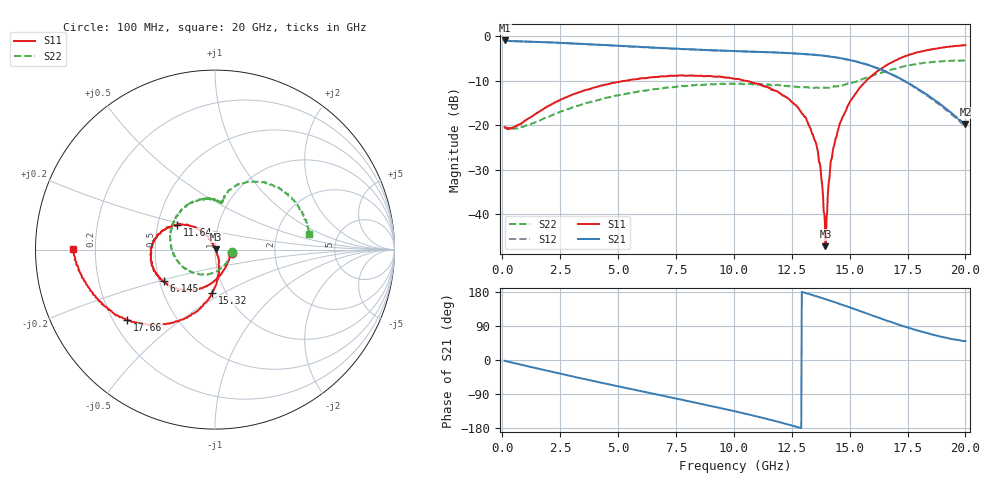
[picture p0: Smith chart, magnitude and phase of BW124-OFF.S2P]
!  2-Port S-parameters saved by WinCal
! VAR MeasName=S-Parameters (CALIBRATED_DATA) read from VNA (N5244A)
! VAR MeasDate=9/14/2012 3:38:30 PM
! VAR NAME=126015-1
! VAR FILENAME=126015-1.S2P
! VAR DATE=9/14/2012 3:38:30 PM
! VAR PHYS_PORTS=1,2
# Hz S MA R 50
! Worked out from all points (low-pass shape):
!   801 points, 100 MHz to 20 GHz, reference 50 ohm
!   highest |S21| = -0.96 dB at 100 MHz (marker M1); lowest = -19.7 dB at 20 GHz (marker M2)
!   |S21| within 3 dB of the highest: start of sweep to 12.9 GHz
!   lowest |S11| = -47.1 dB at 13.96 GHz (marker M3), VSWR 1.01, Z = 50.3 + j0.312 ohm
!   |S11| at or under -10 dB: start of sweep to 5.33 GHz; 10.42192 GHz to 10.4249 GHz (2.98 MHz wide, 0.0286 % of centre); 10.49 GHz to 15.71 GHz (5.216 GHz wide, 39.8 % of centre)
!   |S22| runs from -20.9 to -5.4 dB; largest |S21 - S12| = 0.012
!   S11 on the Smith chart (normalised r, x): 100 MHz: 1.21, -0.04; 6.145 GHz: 0.53, -0.21; 11.64 GHz: 0.63, +0.18; 15.32 GHz: 0.87, -0.44; 17.66 GHz: 0.25, -0.33; 20 GHz: 0.12, +0.00
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1e8  0.09527 -10.2  0.8952 -2.1  0.8914 -2.2  0.09492 -9.2
1.692e9  0.1474 -79.4  0.8581 -24.9  0.8576 -24.9  0.1153 -79.2
3.43325e9  0.2397 -113.7  0.821 -48.7  0.8177 -48.8  0.1715 -129.0
6.144625e9  0.3366 -148.4  0.7532 -84.1  0.7519 -83.9  0.2456 175.9
6.741625e9  0.3505 -155.6  0.7403 -91.8  0.738 -91.7  0.2564 166.0
1.005e10  0.3332 167.7  0.6804 -135.2  0.6803 -135.2  0.2939 114.6
1.1642e10  0.2498 146.9  0.6575 -158.9  0.6583 -158.6  0.2802 95.0
1.27365e10  0.1616 131.2  0.638 -176.7  0.6367 -176.6  0.2681 86.1
1.338325e10  0.07992 119.6  0.6211 171.6  0.6231 171.5  0.2627 82.7
1.365688e10  0.04346 116.2  0.6115 166.5  0.6149 166.3  0.2638 81.6
1.375638e10  0.03046 108.7  0.6091 164.5  0.6105 164.4  0.2649 82.2
1.388075e10  0.01062 87.7  0.6025 162.1  0.6062 161.8  0.2642 82.2
1.395538e10  0.004404 44.7  0.6001 160.5  0.601 160.3  0.2651 81.4
1.403e10  0.01062 -42.1  0.5975 158.9  0.5969 158.8  0.2646 81.3
1.417925e10  0.03833 -66.7  0.59 156.1  0.5917 155.9  0.2683 81.3
1.437825e10  0.06842 -71.5  0.5802 152.2  0.5804 151.7  0.2732 81.8
1.467675e10  0.1213 -79.5  0.562 145.7  0.5618 145.4  0.28 80.6
1.53235e10  0.2403 -93.6  0.5155 131.8  0.5181 131.5  0.3131 78.3
1.669162e10  0.4872 -122.4  0.3849 102.3  0.3867 101.0  0.4147 65.3
1.766175e10  0.6292 -141.3  0.2858 82.8  0.2822 81.0  0.4728 50.2
1.885575e10  0.7354 -163.2  0.1778 63.0  0.1722 61.0  0.5194 29.7
2e10  0.7926 179.6  0.1029 49.7  0.09622 46.5  0.5301 9.6
